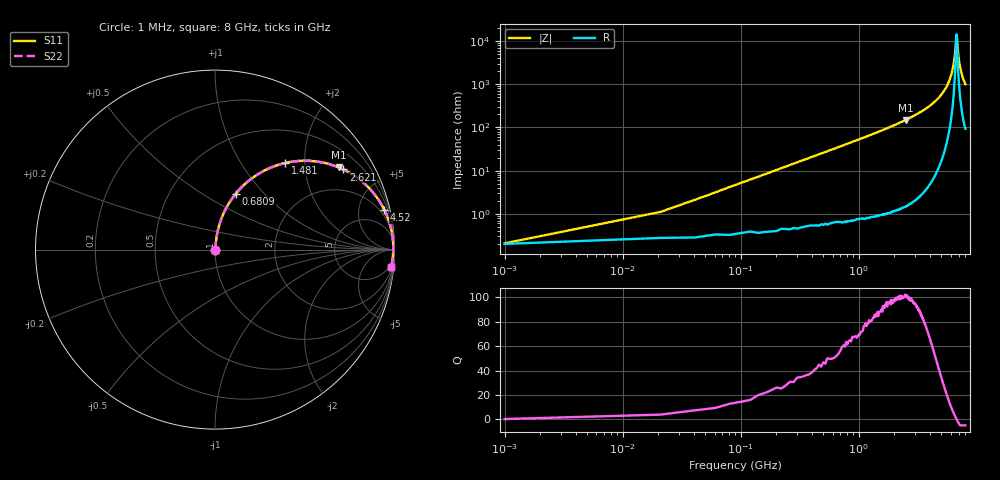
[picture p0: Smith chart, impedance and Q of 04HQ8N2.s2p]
! Coilcraft 0403HQ-8N2 Chip Inductor
! 13 February 2004
# MHZ S MA R 50
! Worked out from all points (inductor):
!   401 points, 1 MHz to 8 GHz, reference 50 ohm
!   read as one part in series: L = 8.15 nH near 40.99 MHz
!   highest Q = 101 at 2.501 GHz (marker M1), where L = 9.5 nH
!   self-resonance near 6.74 GHz
!   S11 on the Smith chart (normalised r, x): 1 MHz: 1.00, +0.00; 680.9 MHz: 1.01, +0.71; 1.481 GHz: 1.02, +1.60; 2.621 GHz: 1.03, +3.18; 4.52 GHz: 1.16, +8.46; 8 GHz: 3, -20
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1  0.002077 14.3  0.998 -0.0  0.998 -0.0  0.002077 14.3
60.992  0.031 82.5  0.996 -1.8  0.996 -1.8  0.031 82.5
100.988  0.052 83.2  0.995 -3.0  0.995 -3.0  0.052 83.2
160.98  0.082 82.5  0.993 -4.7  0.993 -4.7  0.082 82.5
360.955  0.183 77.9  0.978 -10.5  0.978 -10.5  0.183 77.9
680.915  0.332 69.6  0.937 -19.4  0.937 -19.4  0.332 69.6
1340.832  0.581 53.8  0.807 -35.5  0.807 -35.5  0.581 53.8
1480.815  0.622 50.9  0.776 -38.5  0.776 -38.5  0.622 50.9
2500.687  0.827 33.6  0.554 -55.8  0.554 -55.8  0.827 33.6
2620.672  0.843 32.0  0.53 -57.4  0.53 -57.4  0.843 32.0
2680.665  0.85 31.2  0.518 -58.2  0.518 -58.2  0.85 31.2
4000.5  0.95 17.4  0.299 -71.8  0.299 -71.8  0.95 17.4
4520.435  0.969 13.2  0.229 -75.6  0.229 -75.6  0.969 13.2
5340.333  0.986 7.7  0.134 -80.1  0.134 -80.1  0.986 7.7
5920.26  0.991 4.3  0.075 -81.2  0.075 -81.2  0.991 4.3
6240.22  0.993 2.5  0.045 -79.4  0.045 -79.4  0.993 2.5
6500.188  0.993 1.2  0.022 -71.1  0.022 -71.1  0.993 1.2
6680.165  0.993 0.3  0.008639 -36.8  0.008639 -36.8  0.993 0.3
6760.155  0.993 -0.1  0.007187 12.7  0.007187 12.7  0.993 -0.1
7000.125  0.992 -1.2  0.023 69.9  0.023 69.9  0.992 -1.2
7280.09  0.991 -2.5  0.045 77.4  0.045 77.4  0.991 -2.5
8000  0.986 -5.6  0.098 79.1  0.098 79.1  0.986 -5.6
